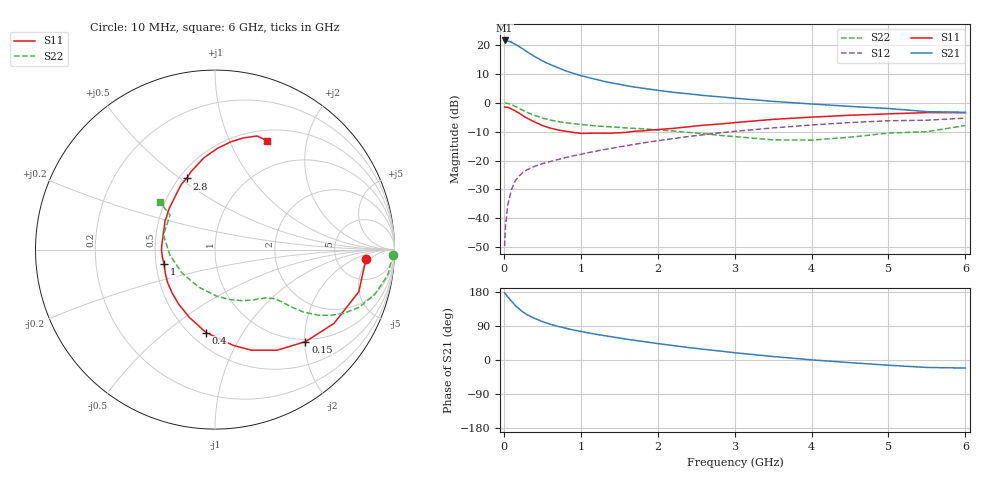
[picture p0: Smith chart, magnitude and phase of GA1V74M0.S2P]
! Infineon Technologies  Discrete & RF Semiconductors
! BF775
! Si NPN RF Bipolar Junction Transistor in SOT23
! VCE = 1.75 V  IC = 4 mA
! Common Emitter S-Parameters:  May  1996
# GHz  S  MA  R  50
!  f  S11  S21  S12  S22
! GHz  MAG  ANG  MAG  ANG  MAG  ANG  MAG  ANG
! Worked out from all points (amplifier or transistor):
!   36 points, 10 MHz to 6 GHz, reference 50 ohm
!   highest |S21| = 21.5 dB at 10 MHz (marker M1)
!   |S21| within 3 dB of that: start of sweep to 251.3 MHz
!   unconditionally stable (mu >= 1): 839.4 MHz to 4.247 GHz; 5.182 GHz to end of sweep
!   at 250 MHz: K = 0.44, MSG = 21.3 dB, |S12| = -24.1 dB
!   at 1.4 GHz: K = 1.15, MAG = 8.9 dB, |S12| = -15.8 dB
!   at 6 GHz: K = 1.01, MAG = 0.5 dB, |S12| = -5.3 dB
!   S11 on the Smith chart (normalised r, x): 10 MHz: 11, -4; 150 MHz: 0.95, -2.02; 400 MHz: 0.60, -0.70; 1 GHz: 0.55, -0.10; 2.8 GHz: 0.55, +0.53; 6 GHz: 0.63, +1.39
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0.01  0.845 -3.4  11.95 177.5  0.0033 87.9  0.9919 -1.6
0.02  0.8369 -6.7  11.82 174.6  0.0069 84.1  0.9857 -3.3
0.05  0.835 -16.3  11.67 167.1  0.017 80.8  0.9735 -8.3
0.1  0.7802 -31.8  11.17 155.0  0.0317 73.6  0.9242 -15.7
0.15  0.7192 -45.5  10.23 143.6  0.045 66.7  0.8639 -21.9
0.2  0.6587 -58.3  9.356 134.5  0.0543 61.8  0.8001 -26.4
0.25  0.5965 -70.0  8.485 126.2  0.0627 57.7  0.7356 -29.9
0.3  0.5428 -79.3  7.643 119.8  0.0689 55.6  0.6823 -32.4
0.4  0.4646 -96.2  6.316 110.0  0.0795 52.3  0.6042 -35.2
0.5  0.4036 -110.8  5.301 101.4  0.0882 51.1  0.5439 -36.6
0.6  0.3651 -123.7  4.601 94.7  0.0958 51.0  0.5021 -37.4
0.7  0.3394 -134.9  4.049 89.0  0.1038 51.0  0.4724 -38.1
0.8  0.3215 -145.3  3.582 84.1  0.1121 51.1  0.4503 -38.7
1  0.295 -163.8  2.953 75.4  0.128 51.8  0.4212 -40.2
1.1  0.2965 -172.2  2.729 71.5  0.137 52.0  0.409 -41.5
1.6  0.3086 156.2  1.96 54.7  0.1817 51.7  0.3661 -48.4
2.2  0.3597 130.4  1.514 38.1  0.2397 48.3  0.325 -61.3
2.8  0.427 111.8  1.267 23.9  0.3005 42.9  0.2736 -79.8
3.5  0.5154 96.9  1.058 9.2  0.3671 34.5  0.2278 -113.3
4.5  0.6073 81.6  0.865 -7.0  0.4539 21.5  0.2534 -173.1
5.5  0.675 69.7  0.702 -19.7  0.4985 6.9  0.3157 142.5
6  0.6728 64.5  0.683 -21.2  0.5409 2.8  0.4039 139.3
